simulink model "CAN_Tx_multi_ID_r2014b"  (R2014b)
settings: Solver=FixedStepDiscrete  StartTime=0.0  StopTime=10.0  RelTol=1e-3
undefined symbols (not defined in the file): bin2dec, bit, identifier, Standard
libraries: etargetslib x2, canmsglib x2, c280xlib x1

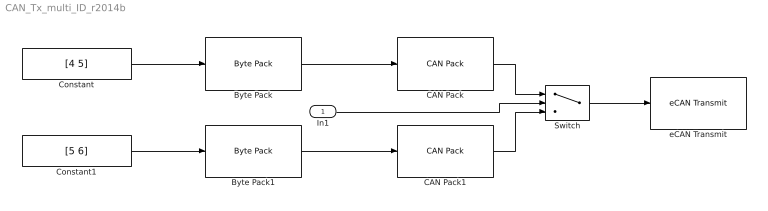
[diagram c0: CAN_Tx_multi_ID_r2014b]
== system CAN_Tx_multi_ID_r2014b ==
  In1 : Inport
  Byte Pack : etargetslib/Byte Pack  datatypes={'uint32'}  byteAlign=1
  Byte Pack1 : etargetslib/Byte Pack  datatypes={'uint32'}  byteAlign=1
  CAN Pack : canmsglib/CAN Pack  MsgList=(none)  MsgName=CAN Msg  MsgIDType=Standard (11-bit identifier)  MsgIdentifier=3  MsgLength=8  NSignals=0  StartBits=0  SignalSizes=0  ByteOrders=0  DataTypes=0  MultiplexTypes=0  MultiplexValues=0  Factors=0  Offsets=0  Minimums=0  Maximums=0  Remote=off
  CAN Pack1 : canmsglib/CAN Pack  MsgList=(none)  MsgName=CAN Msg  MsgIDType=Standard (11-bit identifier)  MsgIdentifier=4  MsgLength=8  NSignals=0  StartBits=0  SignalSizes=0  ByteOrders=0  DataTypes=0  MultiplexTypes=0  MultiplexValues=0  Factors=0  Offsets=0  Minimums=0  Maximums=0  Remote=off
  Constant : Constant  Value=[4 5]  OutDataTypeStr=uint32  SampleTime=-1
  Constant1 : Constant  Value=[5 6]  OutDataTypeStr=uint32  SampleTime=-1
  Switch : Switch
  eCAN Transmit : c280xlib/eCAN Transmit  chipFamily=C280x  useModule=eCAN_A  mailboxNo=1  messageID=bin2dec('111000111')  messageType=Standard (11-bit identifier)  enableBlockingMode=off  postInterrupt=off  interruptLine=0
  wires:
  In1/1 -> Switch/2
  Constant/1 -> Byte Pack/1
  Constant1/1 -> Byte Pack1/1
  CAN Pack/1 -> Switch/1
  CAN Pack1/1 -> Switch/3
  Switch/1 -> eCAN Transmit/1
  Byte Pack/1 -> CAN Pack/1
  Byte Pack1/1 -> CAN Pack1/1
